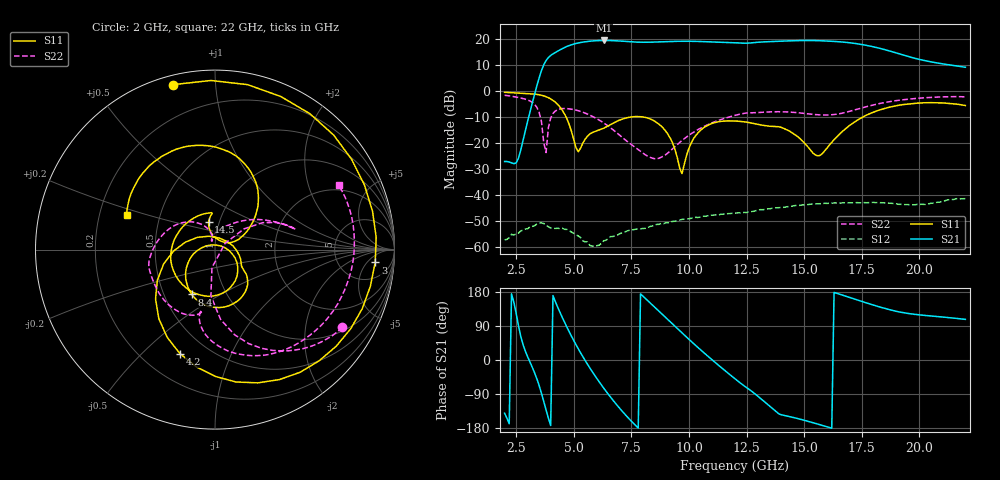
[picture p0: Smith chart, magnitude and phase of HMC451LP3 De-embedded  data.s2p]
! Chelmsford, MA 01824
! http://www.hittite.com
! Tel: 978-250-3343
! Fax: 978-250-3373
! Device  :  HMC451LP3
! Description:  GaAs PHemt MMIC Medium Power AMPLIFIER
! Frequency  :  5 GHz- 18 GHz
! Package  :  LP3  - 3x3 mm Quad Flatpack No-Lead (QFN) Plastic Package: 16 pin
! Ports  :  2 RF, 2 DC
!  Pin  3  = Rfin  = Port 1
!  Pin  10 = Rfout = Port 2
!  Pin  15 = Vdd1
!  Pin  13 = Vdd2
! Voltages:  Vdd1 = Vdd2 = 5.0 Volts
! Currents :  Idd = 120 mA
! Data:  The device was measured on evaluation board 120201-1.
!  Data was collected using a calibrated network analyzer.
!  The evaluation circuit board was modeled and simulated.This was use
!  to removed the evaluation board circuit from the measured data.
!  The reference plane is the center of the package pin.
! Misc:  Lot #
!Date Measured:  03 - 11 -2009
! Date:  03 - 11 -2009
! Note:
!  Hittite Microwave supplies this data as a sample of measured data at the
!  package pin for this package product.  Your particular data for this product
!  may vary.
!  Data was taken at 25 degrees C.
!  Hittite Microwave reserves the right to change this data at anytime.
# MHz S MA R 50
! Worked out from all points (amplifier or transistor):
!   201 points, 2 GHz to 22 GHz, reference 50 ohm
!   highest |S21| = 19.4 dB at 6.3 GHz (marker M1)
!   |S21| within 3 dB of that: 4.534 GHz to 18.27 GHz (13.74 GHz wide, 120 % of centre)
!   unconditionally stable (mu >= 1): start of sweep to end of sweep
!   at 5.3 GHz: K = 31.61, MAG = 19.5 dB, |S12| = -56.3 dB
!   at 12 GHz: K = 10.65, MAG = 19.4 dB, |S12| = -46.9 dB
!   at 22 GHz: K = 5.86, MAG = 14.6 dB, |S12| = -41.3 dB
!   S11 on the Smith chart (normalised r, x): 2 GHz: 0.04, +0.78; 3 GHz: 12, -9; 4.2 GHz: 0.35, -0.66; 8.4 GHz: 0.69, -0.37; 14.5 GHz: 0.89, +0.28; 22 GHz: 0.32, +0.17
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2000  0.9484 104.3  0.04443 -140.5  0.001397 -39.2  0.831 -31.3
3000  0.8955 -4.6  0.2643 8.5  0.00228 -112.2  0.6737 -56.9
3500  0.8487 -46.9  1.795 -67.7  0.002922 -145.6  0.3895 -85.5
3800  0.7797 -72.2  3.868 -132.4  0.002662 -167.9  0.06616 31.8
4200  0.6121 -108.5  5.503 154.4  0.002307 -178.1  0.4137 19.8
4800  0.2307 -178.1  7.48 75.0  0.002106 158.3  0.4564 14.6
5400  0.1015 12.3  8.708 8.3  0.001331 142.4  0.3922 21.9
5800  0.1593 -24.6  9.157 -30.4  0.001059 154.9  0.3284 29.9
6300  0.1937 -35.3  9.369 -74.1  0.001341 171.5  0.2451 42.2
7300  0.3074 -62.6  8.956 -148.4  0.002049 161.4  0.1098 79.4
8400  0.2816 -117.5  8.694 145.9  0.002563 147.0  0.05184 111.7
8700  0.2312 -134.7  8.784 128.7  0.002771 141.1  0.05133 107.5
9600  0.03309 127.5  9.033 77.2  0.003336 123.6  0.1034 105.1
10500  0.1762 -44.1  8.937 27.1  0.003835 103.8  0.1932 127.5
11200  0.2529 -86.2  8.714 -9.5  0.004212 88.9  0.2662 150.5
12000  0.266 -133.7  8.46 -49.7  0.004527 72.4  0.3416 178.4
13100  0.2239 152.5  8.721 -101.0  0.0053 51.7  0.3901 -147.6
13900  0.2067 95.1  9.021 -141.9  0.00578 34.2  0.4016 -124.4
14500  0.1566 103.2  9.248 -151.2  0.006203 42.2  0.3918 -111.5
15400  0.06344 85.3  9.336 -165.7  0.006754 54.1  0.3568 -102.3
18700  0.4901 67.8  5.904 132.9  0.007083 103.6  0.626 -70.8
22000  0.5288 158.5  2.868 107.2  0.008608 177.4  0.7766 27.5
